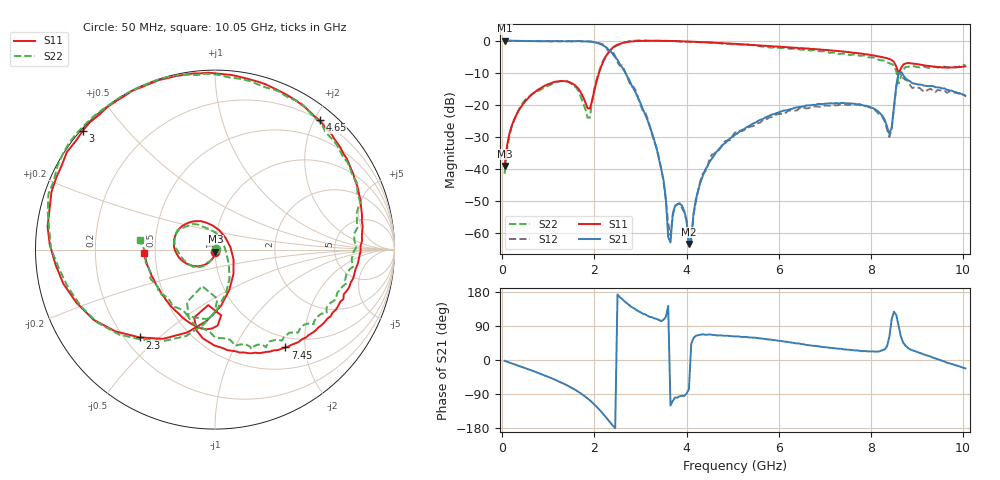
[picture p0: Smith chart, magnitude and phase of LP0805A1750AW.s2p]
! AVX THIN FILM OPERATION
! 0805 Size Low Pass Filter P/N  LP0805A1750AWTR
! Network Analyzer HP8720ES.07.64: Feb 23, 2000 Serial No. US39172382
! Hewlett-Packard
!  2 Feb 2003  04:04:37
! Frequency  S11  S21  S12  S22
# HZ  S  DB R  50
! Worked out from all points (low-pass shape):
!   201 points, 50 MHz to 10.05 GHz, reference 50 ohm
!   highest |S21| = -0.01 dB at 50 MHz (marker M1); lowest = -63.4 dB at 4.05 GHz (marker M2)
!   |S21| within 3 dB of the highest: start of sweep to 2.322 GHz
!   lowest |S11| = -39.1 dB at 50 MHz (marker M3), VSWR 1.02, Z = 50.2 - j1.1 ohm
!   |S11| at or under -10 dB: start of sweep to 2.1 GHz; 8.596838 GHz to 8.604554 GHz (7.716 MHz wide, 0.0897 % of centre)
!   |S22| runs from -41.5 to 0.1 dB; largest |S21 - S12| = 0.061
!   S11 on the Smith chart (normalised r, x): 50 MHz: 1.00, -0.02; 2.3 GHz: 0.26, -0.43; 3 GHz: 0.01, +0.38; 4.65 GHz: 0.20, +2.08; 7.45 GHz: 0.82, -1.63; 10.05 GHz: 0.43, -0.02
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5e7  -39.11 -80.7  -0.01 -2.3  0.05 -2.4  -41.52 14.8
2e8  -26.79 -102.4  -0.02 -8.8  -0.04 -8.7  -26.94 -102.6
5e8  -18.89 -128.6  -0.12 -21.7  -0.08 -21.9  -18.46 -127.6
1.4e9  -12.73 151.1  -0.17 -66.6  -0.19 -66.5  -12.57 152.8
1.75e9  -17.43 95.3  -0.19 -92.0  -0.24 -92.1  -19.33 99.7
1.9e9  -21.18 8.4  -0.30 -106.3  -0.25 -106.9  -24.05 -11.6
2.3e9  -3.81 -130.6  -2.75 -158.9  -3.23 -158.6  -3.81 -128.8
2.6e9  -0.72 178.3  -8.33 161.1  -7.71 162.1  -0.78 179.6
3e9  -0.08 138.1  -19.49 125.8  -20.12 121.1  0.06 140.1
3.4e9  -0.06 111.2  -36.91 105.7  -36.51 102.2  -0.03 112.5
3.55e9  -0.08 102.7  -49.55 113.8  -49.76 111.6  -0.03 104.0
3.6e9  -0.10 100.0  -61.26 142.5  -56.79 138.1  -0.07 101.5
3.85e9  -0.19 87.2  -50.87 -95.5  -50.67 -100.5  -0.25 88.0
4.05e9  -0.29 77.6  -63.40 -76.9  -64.12 -66.6  -0.37 78.0
4.3e9  -0.42 66.3  -44.17 66.8  -43.63 67.1  -0.50 65.9
4.65e9  -0.66 51.0  -34.66 65.0  -34.46 61.2  -0.72 51.1
5.05e9  -0.99 34.6  -29.38 62.4  -28.65 59.1  -1.07 33.5
6.75e9  -2.57 -30.0  -20.02 37.5  -20.57 37.7  -2.92 -29.5
7.45e9  -3.47 -54.4  -19.57 27.6  -20.01 25.9  -4.05 -53.8
8.4e9  -5.74 -93.8  -29.09 61.4  -30.10 61.5  -7.07 -98.7
8.6e9  -10.13 -96.9  -10.10 90.9  -10.30 85.6  -13.34 -109.2
1.005e10  -8.02 -177.0  -17.23 -22.0  -17.02 -16.8  -7.55 172.3
